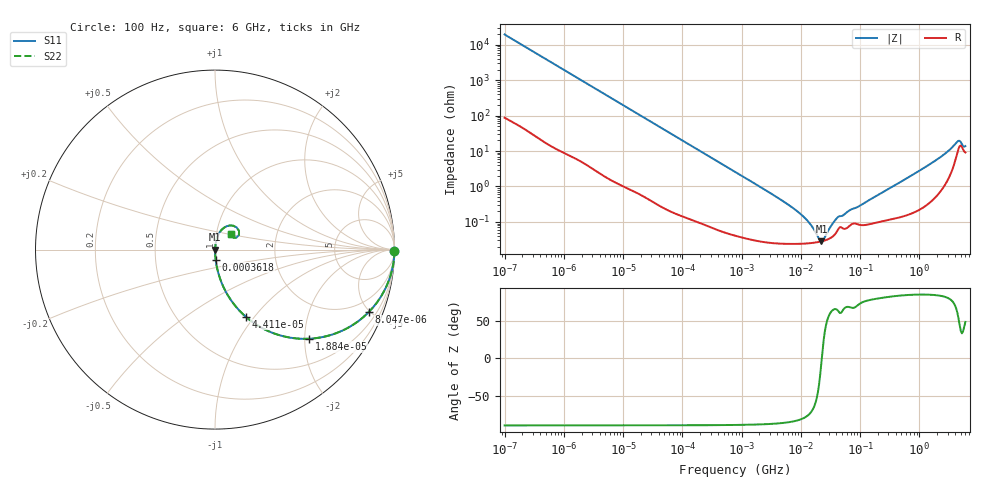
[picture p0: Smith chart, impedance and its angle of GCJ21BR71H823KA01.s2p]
!Murata Part Number: GCJ21BR71H823KA01
!These Parameters are Measured in Series Mode Connection
!Data Generated on Mar 13, 2026
!  o--ll--o
!Port1  Port2
!  o------o
!Operation Temp=25[degC], DC Bias Voltage=0[V]
!Freq. Start=100[Hz] Stop=6[GHz] 401[Steps]
# Hz S RI R 50
!Freq.(Hz) S11(Real) S11(Imag) S21(Real) S21(Imag) S12(Real) S12(Imag) S22(Real) S22(Imag)
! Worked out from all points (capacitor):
!   401 points, 100 Hz to 6 GHz, reference 50 ohm
!   read as one part in series: C = 81.4 nF near 109 Hz
!   lowest |Z| = 28.3 mohm at 22.26 MHz (marker M1)
!   series resonance near 22.58 MHz, so ESL is about 610 pH
!   S11 on the Smith chart (normalised r, x): 100 Hz: open; 8.047 kHz: 1.02, -4.91; 18.84 kHz: 1.01, -2.10; 44.11 kHz: 1.01, -0.90; 361.8 kHz: 1.00, -0.11; 6 GHz: 1.18, +0.21
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100  1 -0.00512  4.91e-05 0.00512  4.91e-05 0.00512  1 -0.00512
2008  0.9892 -0.1009  0.0108 0.1009  0.0108 0.1009  0.9892 -0.1009
4496  0.9497 -0.2161  0.0503 0.2161  0.0503 0.2161  0.9497 -0.2161
8047  0.8566 -0.3481  0.1434 0.3481  0.1434 0.3481  0.8566 -0.3481
18841  0.5252 -0.4965  0.4748 0.4965  0.4748 0.4965  0.5252 -0.4965
40335  0.1968 -0.3947  0.8032 0.3947  0.8032 0.3947  0.1968 -0.3947
44113  0.1703 -0.373  0.8297 0.373  0.8297 0.373  0.1703 -0.373
94437  0.0439 -0.2014  0.9561 0.2014  0.9561 0.2014  0.0439 -0.2014
361830  0.00368 -0.0552  0.9963 0.0552  0.9963 0.0552  0.00368 -0.0552
774597  0.00108 -0.0259  0.9989 0.0259  0.9989 0.0259  0.00108 -0.0259
6948629  0.000246 -0.00264  0.9998 0.00264  0.9998 0.00264  0.000246 -0.00264
1.137099e7  0.000246 -0.00133  0.9998 0.00133  0.9998 0.00133  0.000246 -0.00133
1.555665e7  0.000255 -0.000687  0.9997 0.000687  0.9997 0.000687  0.000255 -0.000687
2.035112e7  0.000273 -0.000188  0.9997 0.000188  0.9997 0.000188  0.000273 -0.000188
2.225763e7  0.000282 -2.56e-05  0.9997 2.56e-05  0.9997 2.56e-05  0.000282 -2.56e-05
2.434276e7  0.000293 0.000137  0.9997 -0.000137  0.9997 -0.000137  0.000293 0.000137
3.330331e7  0.00037 0.000739  0.9996 -0.000739  0.9996 -0.000739  0.00037 0.000739
4.165952e7  0.000575 0.00121  0.9994 -0.00121  0.9994 -0.00121  0.000575 0.00121
3.124326e8  0.00122 0.00871  0.9988 -0.00871  0.9988 -0.00871  0.00122 0.00871
1.873145e9  0.00775 0.053  0.9923 -0.053  0.9923 -0.053  0.00775 0.053
4.385646e9  0.1009 0.1332  0.8991 -0.1332  0.8991 -0.1332  0.1009 0.1332
6e9  0.0917 0.0866  0.9083 -0.0866  0.9083 -0.0866  0.0917 0.0866
